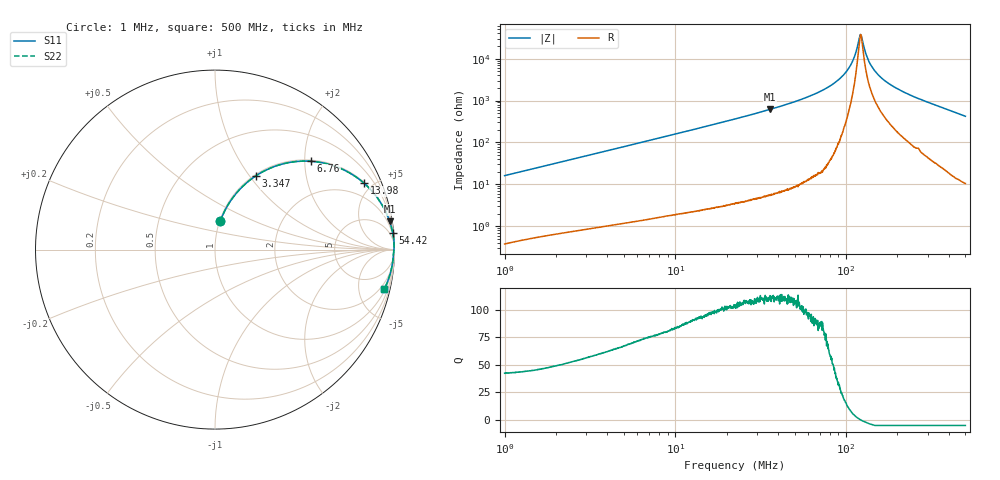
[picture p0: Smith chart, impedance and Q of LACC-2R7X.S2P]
!s-Parameter Generated by FASTRON Sdn. Bhd.
!FASTRON P/N : LACC-2R7X
!Keysight Technologies,E4991B,MY54100416,A.01.15
!Date: Wed Mar 18 09:06:23 2026
!Version  : Rev00 Wed Mar 18 09:06:23 2026
!Data & Calibration Information:
!PortZ  Port1:50+j0  Port2:50+j0
!When reading, reference impedance value at option line is always used.
!Remarks : This data is being provided solely for informational purposes.
!Freq	S11	S21	S12	S22
# Hz S dB R 50
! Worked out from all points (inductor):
!   1601 points, 1 MHz to 500 MHz, reference 50 ohm
!   read as one part in series: L = 2.57 uH near 1.032 MHz
!   highest Q = 112 at 35.78 MHz (marker M1), where L = 2.73 uH
!   self-resonance near 121.6 MHz
!   S11 on the Smith chart (normalised r, x): 1 MHz: 1.01, +0.32; 3.347 MHz: 1.02, +1.07; 6.76 MHz: 1.03, +2.15; 13.98 MHz: 1.05, +4.47; 54.42 MHz: 1, +21; 500 MHz: 1.21, -8.43
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1000000  -15.95 79.5  -0.14 -9.2  -0.14 -9.2  -15.95 79.5
2820919  -7.78 64.9  -0.86 -24.1  -0.86 -24.1  -7.78 64.9
3346665  -6.60 61.1  -1.15 -27.9  -1.15 -27.9  -6.60 61.1
6759791  -2.77 42.6  -3.39 -46.6  -3.39 -46.6  -2.77 42.6
7957584  -2.16 38.1  -4.20 -51.2  -4.20 -51.2  -2.16 38.1
1.397576e7  -0.83 24.0  -7.81 -65.4  -7.81 -65.4  -0.83 24.0
2.236068e7  -0.34 15.3  -11.55 -74.1  -11.55 -74.1  -0.34 15.3
3.577623e7  -0.13 9.3  -15.87 -80.2  -15.87 -80.2  -0.13 9.3
5.442207e7  -0.05 5.4  -20.54 -84.0  -20.54 -84.0  -0.05 5.4
6.307767e7  -0.03 4.3  -22.57 -85.1  -22.57 -85.1  -0.03 4.3
8.214513e7  -0.01 2.4  -27.39 -86.5  -27.39 -86.5  -0.01 2.4
9.821487e7  -0.01 1.3  -32.88 -85.5  -32.88 -85.5  -0.01 1.3
1.090743e8  -0.02 0.7  -38.64 -80.0  -38.64 -80.0  -0.02 0.7
1.192669e8  -0.02 0.1  -49.50 -41.8  -49.50 -41.8  -0.02 0.1
1.216058e8  -0.02 0.0  -51.53 -5.5  -51.53 -5.5  -0.02 0.0
1.244731e8  -0.02 -0.1  -49.11 36.7  -49.11 36.7  -0.02 -0.1
1.33487e8  -0.03 -0.5  -40.23 69.8  -40.23 69.8  -0.03 -0.5
1.414952e8  -0.03 -0.9  -36.19 75.6  -36.19 75.6  -0.03 -0.9
1.559241e8  -0.04 -1.4  -31.94 79.1  -31.94 79.1  -0.04 -1.4
1.77937e8  -0.05 -2.2  -28.15 81.0  -28.15 81.0  -0.05 -2.2
2.543648e8  -0.08 -4.7  -21.63 81.7  -21.63 81.7  -0.08 -4.7
5e8  -0.29 -13.3  -12.79 75.3  -12.79 75.3  -0.29 -13.3
